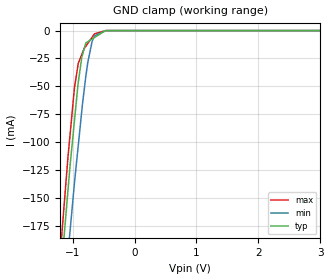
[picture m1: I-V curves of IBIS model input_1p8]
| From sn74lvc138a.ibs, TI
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|   input_1p8 Model
[Model]   input_1p8
Model_type   Input
Vinl = 0.63
Vinh = 1.17
|   typ   min   max
|   (nom PVT)   (fast PVT)   (slow PVT)
|C_comp from frequency sweep method (F=10MHz)
|Average
|C_comp   3.384e-12   3.276e-12   6.749e-12
|C_comp from LC tank measurement(L=1nH)
|Average
|Resonant Frequency(Hz)   3.050e+09   3.060e+09   3.040e+09
C_comp   2.726e-12   2.708e-12   2.744e-12
[Model spec]
|subparameter
Vinl   0.63   0.599   0.662
Vinh   1.17   1.112   1.229
| Where nom  PVT is Nominal Process, 1.8V, 27C
|   Fast PVT is Strong Process,  1.89V, -40C
|   Slow PVT is Weak Process,   1.71V, 125C
[Voltage Range]   1.8   1.71   1.89
|Ambient Temperature   25   85   -40
|Junction Temperature
[Temperature Range]   27   125   -40
[Power Clamp Reference]   1.8   1.71   1.89
[GND Clamp Reference]   0   0   0
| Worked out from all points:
|   GND clamp passes 1 mA (typ) near -0.50 V on its own axis
[GND Clamp]
|   Voltage   I(typ)   I(min)   I(max)
-1.8V     -654.1mA   -675.9mA   -653.6mA
-1.173V   -208.6mA   -261mA     -182.8mA
-1.075V   -144.4mA   -201.4mA   -114.6mA
-1.042V   -122.6mA   -181.2mA   -94.78mA
-967.7mV  -80.02mA   -135.8mA   -50.8mA
-907.2mV  -46.29mA   -102.8mA   -29.3mA
-849.6mV  -23.57mA   -71.41mA   -21.31mA
-755.8mV  -10.13mA   -29.22mA   -11.65mA
-685.7mV  -7.652mA   -9.982mA   -6.103mA
-646.4mV  -6.26mA    -4.781mA   -2.991mA
-471.6mV  -74.99uA   -188.7uA   -53.94uA
3.6V      0A         0A         0A
[POWER Clamp]
|   Voltage   I(typ)   I(min)   I(max)
-1.8V     0A         0A         0A
0V        0A         0A         0A
3.6V      0A         0A         0A
